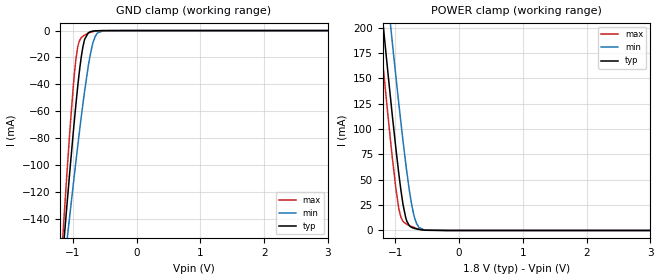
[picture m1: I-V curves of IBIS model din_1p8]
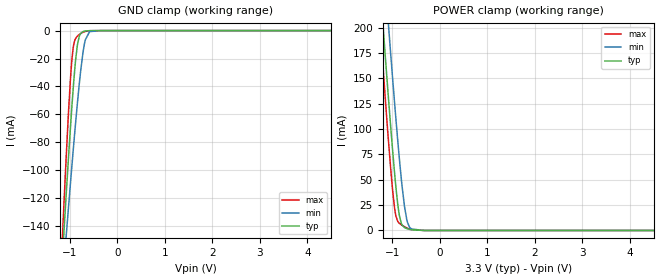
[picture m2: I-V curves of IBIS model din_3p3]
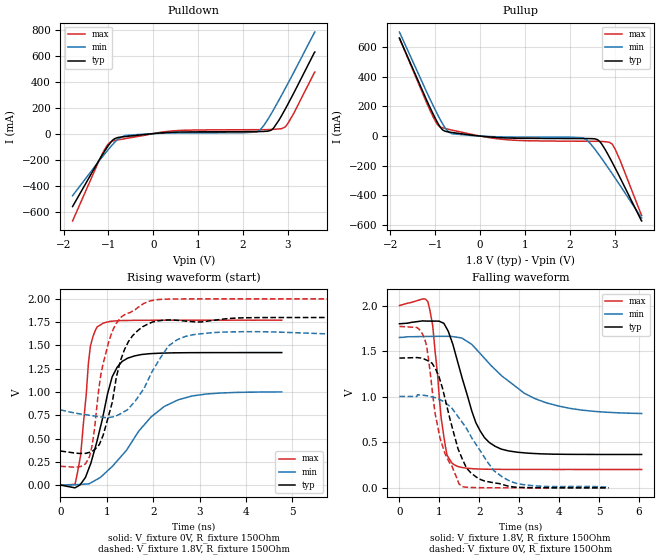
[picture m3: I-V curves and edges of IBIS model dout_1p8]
|Texas Instruments Incorporated
|2-Channel Analog Front-End for Power Monitoring, Control, and Protection
|Marketing part#   Digital Voltage Range   Package-type   #pins
|ADS131A02IPBSR   1.65V-3.6V   TQFP   32
|ADS131A02IPBS   1.65V-3.6V   TQFP   32
[IBIS Ver]   4.1
[File name]   ads131a02.ibs
[File Rev]   1.0
[Date]   8/10/2016
[Source]
| Texas Instruments Incorporated.
| Analog-eLab Design Center, HPA
| 12500 TI Blvd
| Dallas, TX -75243
[Notes]   Revision History:
| Rev 1.0: 8/10/2016
| - Relative Part of ADS131A04
| - Initial version of the model
| - Model generated from simulations in SPECTRE
| - Model matched to SPICE simulation
| - C_comp although listed in numerical order of value are
|   obtained from varying PVT conditions. For PVT conditions for
|   each specific value refer the buffer description under
|   respective [Model]. IBIS model user is responsible for using
|   appropriate C_comp to simulate for Signal Integrity.
|* EXCEPTION:   *
|* - For model dout_*,sclk_*, pullup and pulldown IV tables does not pass *
|*   through 0 because of driver switch(MP36A,MN6) connected to pad.   *
|* - For model xtal1_*,there will be leakage in power and ground clamp   *
|*   IV tables because of resistor R1 connected to pad.   *
|* - For model xtal2_*,pullup and pulldown IV tables does not pass   *
|*   through 0 because of resistors R2<1>, R2<0> connected to pad.   *
[Disclaimer]
| This model is designed as an aid for customers of Texas Instruments.
| TI and its licensors and suppliers make no warranties, either expressed
| or implied, with respect to this  model, including the warranties of
| merchantability or fitness for a particular purpose. The model is
| provided solely on an "as is" basis. The entire risk as to its quality
| and performance is with the customer.
[Copyright]
(C) Copyright 2016 Texas Instruments Incorporated.All rights reserved.
|   ADS131A02IPBS
[Component]   ADS131A02IPBS
[Manufacturer]   TI
[Package]   |32 TQFP- PBS Package
|   typ   min   max
R_pkg   0.0925   0.0458   0.1127
L_pkg   2.0385n   1.7277n   2.3412n
C_pkg   0.4168p   0.3949p   0.5004p
[Pin]  signal_name   model_name   R_pin   L_pin   C_pin
1   AIN1N   nc   0.10434   2.21077n   0.39702p
2   AIN1P   nc   0.10004   2.09233n   0.42617p
3   AIN2N   nc   0.09923   2.03176n   0.40844p
4   AIN2P   nc   0.09868   1.99716n   0.39735p
5   NC   nc   0.09872   1.99814n   0.39743p
6   NC   nc   0.09946   2.03744n   0.40887p
7   NC   nc   0.10038   2.10094n   0.42678p
8   NC   nc   0.10490   2.22492n   0.39763p
9   AVDD   power   0.06167   1.99066n   0.43472p
10   AVSS   gnd   0.04584   1.81954n   0.50035p
11   VNCP   nc   0.05877   1.79195n   0.45455p
12   REFP   nc   0.09782   1.98852n   0.40436p
13   REFN   nc   0.09770   1.98667n   0.40459p
14   REFEXT   nc   0.10114   2.06673n   0.41324p
15   IOVDD   power   0.10037   2.10352n   0.42705p
16   RESV   power   0.10608   2.24459n   0.40003p
17   _RESET   din   0.10273   2.19143n   0.39487p
18   _DONE   dout   0.09860   2.07366n   0.42585p
19   _DRDY   sclk   0.09685   1.99682n   0.40719p
20   DIN   din   0.09731   1.97621n   0.39759p
21   DOUT   dout   0.09886   1.99951n   0.39927p
22   SCLK   sclk   0.10136   2.06459n   0.41213p
23   _CS   din   0.10590   2.18322n   0.43392p
24   NC   nc   0.11269   2.34124n   0.40456p
25   XTAL1/CLKIN   xtal1   0.10082   2.15621n   0.39548p
26   XTAL2   xtal2   0.09605   2.02922n   0.42626p
27   GND   gnd   0.05705   1.74326n   0.44120p
28   CAP   nc   0.05750   1.72774n   0.43775p
29   IOVDD   power   0.05823   1.75365n   0.43078p
30   M0   din   0.09686   1.99257n   0.40576p
31   M1   din   0.09979   2.08693n   0.42778p
32   M2   din   0.10552   2.22902n   0.39817p
|   Model Selectors
[Model Selector] din
din_1p8   1.8V   digital Input
din_3p3   3.3V   digital Input
[Model Selector] dout
dout_1p8   1.8V   digital Output
dout_3p3   3.3V   digital Output
[Model Selector] sclk
sclk_1p8   1.8V   digital IO
sclk_3p3   3.3V   digital IO
[Model Selector] xtal1
xtal1_1p8   1.8V   digital Input
xtal1_3p3   3.3V   digital Input
[Model Selector] xtal2
xtal2_1p8   1.8V   digital Output
xtal2_3p3   3.3V   digital Output
| Models and submodels in the file (10): din_1p8 (Input), din_3p3 (Input), dout_1p8 (Output), dout_3p3 (Output), sclk_1p8 (I/O), sclk_3p3 (I/O), xtal1_1p8 (Input), xtal1_3p3 (Input), xtal2_1p8 (Output), xtal2_3p3 (Output)
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|   din_1p8 Model
[Model]   din_1p8
Model_type   Input
Vinl = 0.36
Vinh = 1.44
|   typ   min   max
|   (nom PVT)   (fast PVT)   (slow PVT)
C_comp   1.601e-12   1.593e-12   1.601e-12
| Where nom  PVT is Nominal Process, 1.8V, 27C
|   Fast PVT is Strong Process,  2V, -40C
|   Slow PVT is Weak Process,   1.65V, 125C
[Voltage Range]   1.8   1.65   2
|Junction Temperature
[Temperature Range]   27   125   -40
[Power Clamp Reference]   1.8   1.65   2
[GND Clamp Reference]   0   0   0
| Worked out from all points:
|   GND clamp passes 1 mA (typ) near -0.73 V on its own axis
|   POWER clamp passes 1 mA (typ) near -0.63 V on its own axis
[GND Clamp]
|   Voltage   I(typ)   I(min)   I(max)
-1.8V     -554.1mA   -474.7mA   -657.7mA
-1.148V   -160.7mA   -180.1mA   -145.4mA
-1.106V   -136.7mA   -161.9mA   -114.9mA
-1.055V   -108.2mA   -139.9mA   -79.28mA
-994mV    -75.58mA   -114.3mA   -41.37mA
-952.2mV  -54.57mA   -97.05mA   -21.15mA
-902mV    -31.92mA   -76.95mA   -8.255mA
-844.2mV  -12.3mA    -54.95mA   -4.252mA
-750.6mV  -1.393mA   -23.99mA   -1.807mA
-651.6mV  -214.4uA   -4.487mA   -445.2uA
-522.9mV  -14.93uA   -149.5uA   -26.28uA
3.6V      0A         0A         0A
[POWER Clamp]
|   Voltage   I(typ)   I(min)   I(max)
-1.8V     611.3mA    673.1mA    583.4mA
-1.411V   346.4mA    415.3mA    309.4mA
-1.208V   213.2mA    284.8mA    172.3mA
-1.168V   187.7mA    259.7mA    146.3mA
-1.069V   126mA      198.2mA    84.14mA
-989.9mV  79.46mA    150.4mA    40.13mA
-928.8mV  47.09mA    115mA      16.48mA
-838mV    12.59mA    66.16mA    6.746mA
-752.4mV  3.285mA    28.24mA    4.044mA
-668.1mV  1.506mA    6.791mA    2.06mA
-521.2mV  219.2uA    354.5uA    240.9uA
3.6V      0A         0A         0A
|   din_3p3 Model
[Model]   din_3p3
Model_type   Input
Vinl = 0.66
Vinh = 2.64
|   typ   min   max
|   (nom PVT)   (fast PVT)   (slow PVT)
C_comp   1.546e-12   1.546e-12   1.561e-12
| Where nom  PVT is Nominal Process, 3.3V, 27C
|   Fast PVT is Strong Process,  3.6V, -40C
|   Slow PVT is Weak Process,   3V, 125C
[Voltage Range]   3.3   3   3.6
|Junction Temperature
[Temperature Range]   27   125   -40
[Power Clamp Reference]   3.3   3   3.6
[GND Clamp Reference]   0   0   0
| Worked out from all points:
|   GND clamp passes 1 mA (typ) near -0.73 V on its own axis
|   POWER clamp passes 1 mA (typ) near -0.63 V on its own axis
[GND Clamp]
|   Voltage   I(typ)   I(min)   I(max)
-3.3V     -1.489A    -1.173A    -1.877A
-1.197V   -188.2mA   -201mA     -180.7mA
-1.115V   -140.9mA   -165.1mA   -120mA
-1.076V   -118.9mA   -148.3mA   -92.5mA
-985.2mV  -70.27mA   -110.1mA   -35.72mA
-924mV    -40.72mA   -85.13mA   -11.88mA
-838.2mV  -10.5mA    -52.28mA   -3.986mA
-720mV    -732.9uA   -15.72mA   -1.234mA
-672mV    -304.1uA   -6.767mA   -613.8uA
-582mV    -52.5uA    -738.4uA   -104.3uA
-330mV    -89.41nA   -746.6nA   -56.53nA
6.6V      0A         0A         0A
[POWER Clamp]
|   Voltage   I(typ)   I(min)   I(max)
-3.3V     1.672A     1.701A     1.679A
-1.274V   254.9mA    325.9mA    215.1mA
-1.151V   175.7mA    247.9mA    134mA
-1.086V   135.4mA    207.7mA    93.34mA
-990mV    78.71mA    149.7mA    39.42mA
-920.4mV  42.32mA    109.5mA    14.15mA
-861mV    18.45mA    77.22mA    7.689mA
-808.5mV  7.107mA    51.21mA    5.653mA
-693mV    1.863mA    10.79mA    2.546mA
-597mV    682.7uA    1.477mA    880.6uA
-330mV    2.194uA    7.268uA    1.05uA
6.6V      0A         0A         0A
|   dout_1p8 Model
[Model]   dout_1p8
Model_type   Output
Polarity   Non-Inverting
Vmeas = 0.9
Vref = 0
Cref = 2pF
Rref = 150
|   typ   min   max
|   (nom PVT)   (fast PVT)   (slow PVT)
C_comp   1.650e-12   1.625e-12   1.747e-12
| Where nom  PVT is Nominal Process, 1.8V, 27C
|   Fast PVT is Strong Process,  2V, -40C
|   Slow PVT is Weak Process,   1.65V, 125C
[Voltage Range]   1.8   1.65   2
|Junction Temperature
[Temperature Range]   27   125   -40
[Pullup Reference]   1.8   1.65   2
[Pulldown Reference]   0   0   0
[Power Clamp Reference]   1.8   1.65   2
[GND Clamp Reference]   0   0   0
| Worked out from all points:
|   slope of the pulldown table from 0 to 0.27 V, typ, clamps not added: 34.9 ohm
|   slope of the pullup table from 0 to 0.27 V, typ, clamps not added: 37.2 ohm
|   falling waveform, V_fixture 1.8V, R_fixture 150Ohm: 20-80 % time 612ps typ, 1.38ns min, 251ps max; typ from 1.8 V to 0.366 V
|   rising waveform, V_fixture 0V, R_fixture 150Ohm: 20-80 % time 418ps typ, 1.01ns min, 187ps max; typ from 0 V to 1.42 V
|   rising waveform, V_fixture 1.8V, R_fixture 150Ohm: 20-80 % time 451ps typ, 595ps min, 390ps max; typ from 0.366 V to 1.8 V
|   falling waveform, V_fixture 0V, R_fixture 150Ohm: 20-80 % time 562ps typ, 906ps min, 440ps max; typ from 1.42 V to 0 V
[Pulldown]
|   Voltage   I(typ)   I(min)   I(max)
-1.8V     -561.5mA   -477.8mA   -672.6mA
-1.109V   -147.5mA   -166.8mA   -137.1mA
-1.01V    -95.21mA   -125.1mA   -81.69mA
-914.4mV  -53.71mA   -86.63mA   -57.35mA
-631.8mV  -22.97mA   -14.43mA   -38.99mA
468mV     10.98mA    4.902mA    21.86mA
1.98V     14.93mA    6.5mA      29.81mA
2.379V    15.81mA    28.17mA    30.2mA
2.666V    37.2mA     174.7mA    32.54mA
2.936V    184.9mA    343.3mA    50.16mA
3.136V    314.9mA    473.7mA    158.9mA
3.6V      628.5mA    781.8mA    474.2mA
[Pullup]
|   Voltage   I(typ)   I(min)   I(max)
-1.8V     659.9mA    701.2mA    659.5mA
-1.194V   242.3mA    297.4mA    225.1mA
-986.4mV  110.9mA    167mA      93.37mA
-848mV    44.82mA    87.82mA    56.5mA
-701.1mV  27.39mA    27.04mA    45.23mA
574.2mV   -12.58mA   -6.351mA   -24.2mA
2.292V    -16.8mA    -11.84mA   -34.94mA
2.617V    -24.32mA   -112.6mA   -35.58mA
2.724V    -60.21mA   -157.7mA   -36.84mA
2.952V    -182.3mA   -257.8mA   -58.34mA
3.124V    -283.6mA   -335.3mA   -166.6mA
3.6V      -572.6mA   -552.7mA   -535.3mA
[Ramp]
R_load = 150
|   typ   min   max
dV/dt_r   0.854094/4.3723e-10   0.601056/1.00694e-09   1.06268/2.08709e-10
dV/dt_f   0.860507/6.21652e-10   0.503076/1.3733e-09   1.07897/2.61361e-10
[Falling Waveform]
V_fixture = 1.8V
V_fixture_min = 1.65V
V_fixture_max = 2V
R_fixture = 150Ohm
|   Time   V(typ)   V(min)   V(max)
0s        1.8V       1.65V      2V
714.2ps   1.829V     1.661V     2.042V
835.1ps   1.829V     1.662V     1.776V
1.097ns   1.808V     1.662V     612.3mV
1.192ns   1.743V     1.662V     361.2mV
1.321ns   1.596V     1.66V      269mV
1.915ns   715.6mV    1.526V     208.2mV
2.396ns   456.4mV    1.3V       203.1mV
3.674ns   371.6mV    933.9mV    201.9mV
6.07ns    366.1mV    815.5mV    201.8mV
[Rising Waveform]
V_fixture = 0V
V_fixture_min = 0V
V_fixture_max = 0V
R_fixture = 150Ohm
|   Time   V(typ)   V(min)   V(max)
0s        1.048nV    65.85nV    185.3pV
314.2ps   -29.52mV   3.114mV    7.652mV
435.1ps   10.08mV    7.188mV    319mV
645.1ps   221.1mV    21.39mV    1.49V
791.8ps   480.6mV    62.55mV    1.699V
1.115ns   1.163V     199.3mV    1.76V
1.452ns   1.364V     395.6mV    1.768V
1.954ns   1.412V     731.6mV    1.77V
2.534ns   1.421V     915.1mV    1.771V
4.77ns    1.423V     1.001V     1.771V
[Rising Waveform]
V_fixture = 1.8V
V_fixture_min = 1.65V
V_fixture_max = 2V
R_fixture = 150Ohm
|   Time   V(typ)   V(min)   V(max)
0s        365.9mV    807.4mV    201.7mV
629.5ps   351.9mV    749.3mV    309.6mV
736.7ps   382.1mV    741.5mV    611mV
837.6ps   435mV      734mV      1.072V
1.091ns   841.3mV    729.2mV    1.614V
1.378ns   1.453V     789.8mV    1.828V
1.945ns   1.743V     1.188V     1.98V
2.516ns   1.77V      1.561V     1.999V
3.289ns   1.769V     1.637V     2V
13.27ns   1.8V       1.65V      2V
[Falling Waveform]
V_fixture = 0V
V_fixture_min = 0V
V_fixture_max = 0V
R_fixture = 150Ohm
|   Time   V(typ)   V(min)   V(max)
0s        1.423V     1.003V     1.771V
620.9ps   1.413V     1.014V     1.648V
678.7ps   1.402V     1.011V     1.564V
896.5ps   1.311V     988.8mV    811mV
1.014ns   1.186V     968.1mV    550.4mV
1.555ns   338.4mV    730.1mV    19.78mV
1.917ns   121.2mV    478mV      2.608mV
2.372ns   55.55mV    186.8mV    699.5uV
2.789ns   14.02mV    68.75mV    290.2uV
5.241ns   92.94uV    7.99mV     8.231uV
